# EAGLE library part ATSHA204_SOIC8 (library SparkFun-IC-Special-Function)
Crypto 4.5KB I2C Datasheet SparkFun Products CryptoCape (DEV-12773) SparkFun CryptoShield (DEV-13183)
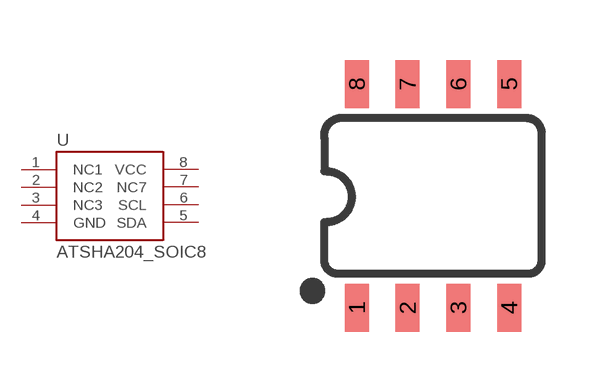
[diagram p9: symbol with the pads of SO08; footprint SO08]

Designator prefix U

## ATSHA204_SOIC8 (PROD_ID: IC-11981; VALUE: ATSHA204)  [SO08]
1  NC1  nc
2  NC2  nc
3  NC3  nc
4  GND  pwr
5  SDA
6  SCL
7  NC7  nc
8  VCC  pwr

## Footprint SO08 (pad centres in mm)
SOIC, 0.15 inch width
smd 0.6 x 1.2: 1 -1.905,-2.8; 2 -0.635,-2.8; 3 0.635,-2.8; 4 1.905,-2.8; 5 1.905,2.8; 6 0.635,2.8; 7 -0.635,2.8; 8 -1.905,2.8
